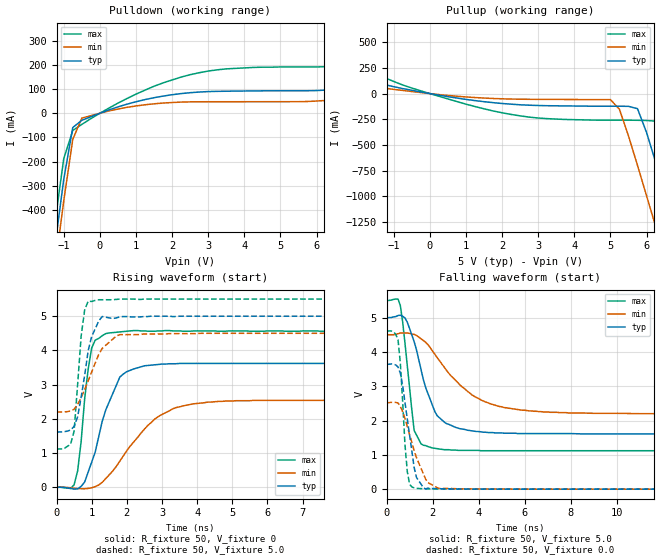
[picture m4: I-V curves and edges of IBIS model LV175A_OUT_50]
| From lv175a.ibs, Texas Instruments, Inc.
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|   Model LV175A_OUT_50
[Model]   LV175A_OUT_50
Model_type  Output
Polarity   Non-Inverting
Vmeas = 2.50v
Cref = 15pf
| variable   typ   min   max
C_comp   4.62pf   3.47pf   5.77pf
[Temperature Range]   25   85   -40
[Voltage Range]   5.0   4.5   5.5
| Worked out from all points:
|   slope of the pulldown table from 0 to 0.75 V, typ, clamps not added: 19.9 ohm
|   slope of the pullup table from 0 to 0.75 V, typ, clamps not added: 17.2 ohm
|   rising waveform, R_fixture 50, V_fixture 0: 20-80 % time 669ps typ, 1.22ns min, 282ps max; typ from 0 V to 3.62 V
|   falling waveform, R_fixture 50, V_fixture 5.0: 20-80 % time 895ps typ, 1.95ns min, 410ps max; typ from 5 V to 1.61 V
|   rising waveform, R_fixture 50, V_fixture 5.0: 20-80 % time 339ps typ, 572ps min, 201ps max; typ from 1.61 V to 5 V
|   falling waveform, R_fixture 50, V_fixture 0.0: 20-80 % time 457ps typ, 747ps min, 251ps max; typ from 3.64 V to 0 V
[Pulldown]
|   Voltage   I(typ)   I(min)   I(max)
-5V       -5.14A     -5.22A     -5.05A
-1.25V    -557mA     -649mA     -461mA
-1V       -274mA     -363mA     -188mA
-750mV    -58.9mA    -108mA     -71.3mA
-500mV    -29.2mA    -20mA      -46.2mA
0V        -3.33nA    -3.4nA     -3.57nA
1.25V     56.7mA     35.2mA     96mA
2.5V      85.3mA     47.3mA     160mA
3.5V      91.4mA     47.8mA     184mA
7V        108mA      63mA       206mA
8.25V     142mA      85.5mA     255mA
10V       202mA      122mA      357mA
[Pullup]
|   Voltage   I(typ)   I(min)   I(max)
-5V       348mA      197mA      640mA
-750mV    48.6mA     30.8mA     83.5mA
1.25V     -68.2mA    -38.5mA    -126mA
3V        -116mA     -56.1mA    -238mA
5V        -123mA     -58.9mA    -259mA
5.25V     -123mA     -153mA     -259mA
5.75V     -147mA     -699mA     -260mA
6.25V     -664mA     -1.29A     -268mA
6.5V      -960mA     -1.6A      -403mA
6.75V     -1.26A     -1.9A      -685mA
7.25V     -1.87A     -2.51A     -1.28A
10V       -5.25A     -5.89A     -4.66A
[Ramp]
| variable   typ   min   max
dV/dt_r   2.18E+00/5.97E-10   1.54E+00/1.23E-09   2.74E+00/2.58E-10
dV/dt_f   2.08E+00/8.86E-10   1.41E+00/1.96E-09   2.66E+00/3.41E-10
R_load = 50
[Rising Waveform]
R_fixture = 50
V_fixture = 0
|   Time   V(typ)   V(min)   V(max)
0s        0V         0V         0V
500ps     -54.4mV    -28mV      73.1mV
600ps     -46mV      -37.3mV    478mV
800ps     155mV      -41.6mV    2.59V
1ns       736mV      -13.7mV    4.07V
1.5ns     2.5V       366mV      4.51V
2ns       3.38V      1.07V      4.56V
2.9ns     3.59V      2.07V      4.57V
4.3ns     3.62V      2.49V      4.57V
25ns      3.62V      2.54V      4.56V
[Falling Waveform]
R_fixture = 50
V_fixture = 5.0
V_fixture_min = 4.5
V_fixture_max = 5.5
|   Time   V(typ)   V(min)   V(max)
0s        5V         4.5V       5.5V
600ps     5.07V      4.55V      5.35V
900ps     4.87V      4.55V      3.61V
1.2ns     4.3V       4.51V      1.71V
1.5ns     3.48V      4.38V      1.32V
2ns       2.43V      4.02V      1.2V
2.6ns     1.91V      3.47V      1.15V
3.7ns     1.7V       2.75V      1.13V
5.9ns     1.62V      2.3V       1.12V
25ns      1.61V      2.2V       1.12V
[Rising Waveform]
R_fixture = 50
V_fixture = 5.0
V_fixture_min = 4.5
V_fixture_max = 5.5
|   Time   V(typ)   V(min)   V(max)
0s        1.61V      2.2V       1.12V
400ps     1.67V      2.23V      1.26V
500ps     1.78V      2.28V      1.64V
700ps     2.63V      2.62V      4.42V
800ps     3.27V      2.86V      5.18V
900ps     3.99V      3.11V      5.44V
1ns       4.41V      3.37V      5.43V
1.3ns     4.99V      4.06V      5.48V
1.8ns     4.98V      4.46V      5.5V
25ns      5V         4.5V       5.5V
[Falling Waveform]
R_fixture = 50
V_fixture = 0.0
|   Time   V(typ)   V(min)   V(max)
0s        3.64V      2.53V      4.61V
500ps     3.56V      2.51V      4.35V
600ps     3.38V      2.41V      3.67V
800ps     2.53V      2.06V      1.3V
900ps     2.05V      1.83V      523mV
1ns       1.58V      1.59V      144mV
1.2ns     629mV      1.12V      38.1mV
1.6ns     43mV       447mV      12.4mV
2.3ns     12.9mV     21.1mV     4.5mV
25ns      0V         0V         7.74uV
